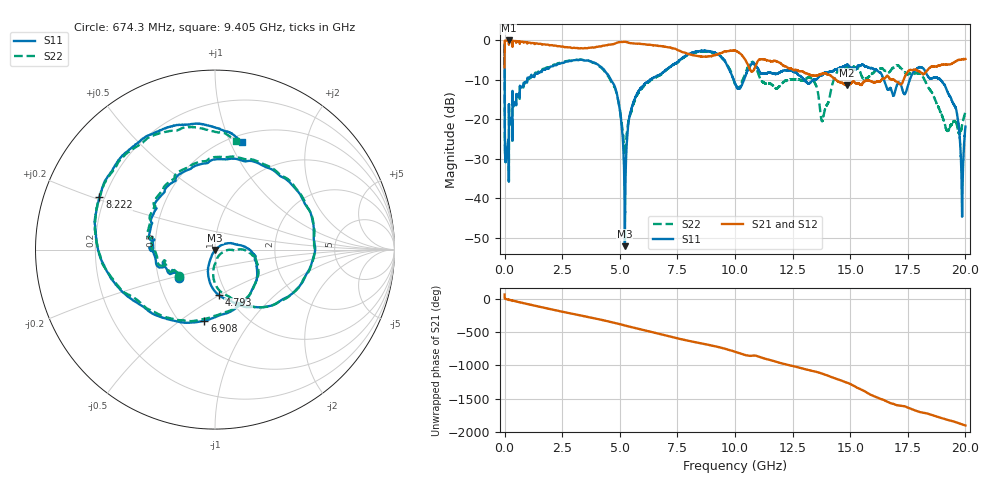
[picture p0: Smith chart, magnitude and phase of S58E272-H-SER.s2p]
!{S58E272}
!Johanson Technology Inc.
!www.johansontechnology.com
!Test Board Conditions:
!Substrate Type  RO4350B
!Substrate Thickness  60 mil
!Substrate Dk  3.66
!TL Type: GCPW
!TL Trace Width  115 mil
!TL Gap  52 mil
!Electrode orientation  Horizontal
!DUT TOPOLOGY	SERIES
!Mounting Pad LxW  55x428 mil
! Created Wed Apr 14 11:39:25 2021
# mhz S ma R 50
! 2 Port Network Data from SP1.SP block
! freq  magS11  angS11  magS21  angS21  magS12  angS12  magS22  angS22
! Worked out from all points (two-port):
!   20001 points, 300 kHz to 20 GHz, reference 50 ohm
!   highest |S21| = -0.02 dB at 183.3 MHz (marker M1); lowest = -11.4 dB at 14.86 GHz (marker M2)
!   |S21| within 3 dB of the highest: 939.4 kHz to 7.756 GHz (7.755 GHz wide, 200 % of centre); 9.474 GHz to 10.15 GHz (673.8 MHz wide, 6.87 % of centre)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
!   lowest |S11| = -52.2 dB at 5.221 GHz (marker M3), VSWR 1.00, Z = 50.2 - j0.195 ohm
!   |S11| at or under -10 dB: 4.615 GHz to 6.321 GHz (1.705 GHz wide, 31.2 % of centre); 16.46 GHz to 17.58 GHz (1.124 GHz wide, 6.6 % of centre); 18.92 GHz to end of sweep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
!   |S22| runs from -35.7 to -1.0 dB; largest |S21 - S12| = 0.0077
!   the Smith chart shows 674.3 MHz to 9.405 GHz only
!   S11 on the Smith chart (normalised r, x): 674.3 MHz: 0.63, -0.21; 4.793 GHz: 0.91, -0.50; 6.908 GHz: 0.66, -0.62; 8.222 GHz: 0.18, +0.21; 9.405 GHz: 0.57, +1.10
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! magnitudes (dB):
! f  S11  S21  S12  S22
! 300 kHz  -1.0  -6.8  -6.9  -1.0
! 102.3 MHz  -27.8  -0.1  -0.1  -27.9
! 183.3 MHz  -30.1  0.0  0.0  -30.4
! 674.3 MHz  -11.8  -0.3  -0.3  -12.0
! 3.334 GHz  -4.9  -2.0  -2.0  -4.9
! 4.793 GHz  -11.9  -0.8  -0.8  -12.2
! 5.221 GHz  -52.2  -0.4  -0.4  -28.5
! 5.618 GHz  -15.3  -0.8  -0.8  -15.7
! 6.667 GHz  -8.8  -1.4  -1.4  -9.0
! 6.908 GHz  -7.9  -1.6  -1.6  -8.1
! 8.222 GHz  -3.0  -3.8  -3.8  -3.1
! 9.405 GHz  -4.2  -3.2  -3.2  -4.2
! 10 GHz  -10.9  -2.6  -2.6  -11.1
! 10.74 GHz  -5.8  -7.9  -7.9  -5.5
! 13.33 GHz  -10.3  -8.9  -8.9  -9.8
! 13.8 GHz  -8.8  -8.5  -8.5  -20.4
! 14.86 GHz  -6.2  -11.4  -11.4  -6.8
! 16.67 GHz  -12.5  -9.3  -9.4  -8.1
! 18.12 GHz  -6.9  -8.4  -8.5  -8.9
! 19.53 GHz  -16.5  -5.5  -5.5  -20.5
! 19.85 GHz  -41.1  -4.8  -4.8  -21.7
! 20 GHz  -21.9  -4.7  -4.7  -18.0
